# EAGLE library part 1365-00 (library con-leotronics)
DUAL ROW STRAIGHT HEADER 1364 SERIES. 1.27mm x 1.27mm. Without Fixing Post. SMT Source: http://www.leotronics.co.uk/Conexcon/Data%20Sheets/sec.%20A/1364ing.pdf
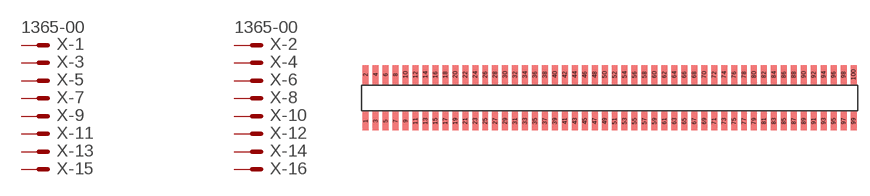
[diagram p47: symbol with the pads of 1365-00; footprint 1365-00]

Designator prefix X; gates -1=MVAL -2=MVAL -3=M -4=M -5=M -6=M -7=M -8=M -9=M -10=M -11=M -12=M -13=M -14=M -15=M -16=M -17=M -18=M -19=M -20=M -21=M -22=M -23=M -24=M -25=M -26=M -27=M -28=M -29=M -30=M -31=M -32=M -33=M -34=M -35=M -36=M -37=M -38=M -39=M -40=M -41=M -42=M -43=M -44=M -45=M -46=M -47=M -48=M -49=M -50=M -51=M -52=M -53=M -54=M -55=M -56=M -57=M -58=M -59=M -60=M -61=M -62=M -63=M -64=M -65=M -66=M -67=M -68=M -69=M -70=M -71=M -72=M -73=M -74=M -75=M -76=M -77=M -78=M -79=M -80=M -81=M -82=M -83=M -84=M -85=M -86=M -87=M -88=M -89=M -90=M -91=M -92=M -93=M -94=M -95=M -96=M -97=M -98=M -99=M -100=M

## 1365-00 (OC_FARNELL: unknown; OC_NEWARK: unknown)  [1365-00]
1  -1:S  pas
2  -2:S  pas
3  -3:S  pas
4  -4:S  pas
5  -5:S  pas
6  -6:S  pas
7  -7:S  pas
8  -8:S  pas
9  -9:S  pas
10  -10:S  pas
11  -11:S  pas
12  -12:S  pas
13  -13:S  pas
14  -14:S  pas
15  -15:S  pas
16  -16:S  pas
17  -17:S  pas
18  -18:S  pas
19  -19:S  pas
20  -20:S  pas
21  -21:S  pas
22  -22:S  pas
23  -23:S  pas
24  -24:S  pas
25  -25:S  pas
26  -26:S  pas
27  -27:S  pas
28  -28:S  pas
29  -29:S  pas
30  -30:S  pas
31  -31:S  pas
32  -32:S  pas
33  -33:S  pas
34  -34:S  pas
35  -35:S  pas
36  -36:S  pas
37  -37:S  pas
38  -38:S  pas
39  -39:S  pas
40  -40:S  pas
41  -41:S  pas
42  -42:S  pas
43  -43:S  pas
44  -44:S  pas
45  -45:S  pas
46  -46:S  pas
47  -47:S  pas
48  -48:S  pas
49  -49:S  pas
50  -50:S  pas
51  -51:S  pas
52  -52:S  pas
53  -53:S  pas
54  -54:S  pas
55  -55:S  pas
56  -56:S  pas
57  -57:S  pas
58  -58:S  pas
59  -59:S  pas
60  -60:S  pas
61  -61:S  pas
62  -62:S  pas
63  -63:S  pas
64  -64:S  pas
65  -65:S  pas
66  -66:S  pas
67  -67:S  pas
68  -68:S  pas
69  -69:S  pas
70  -70:S  pas
71  -71:S  pas
72  -72:S  pas
73  -73:S  pas
74  -74:S  pas
75  -75:S  pas
76  -76:S  pas
77  -77:S  pas
78  -78:S  pas
79  -79:S  pas
80  -80:S  pas
81  -81:S  pas
82  -82:S  pas
83  -83:S  pas
84  -84:S  pas
85  -85:S  pas
86  -86:S  pas
87  -87:S  pas
88  -88:S  pas
89  -89:S  pas
90  -90:S  pas
91  -91:S  pas
92  -92:S  pas
93  -93:S  pas
94  -94:S  pas
95  -95:S  pas
96  -96:S  pas
97  -97:S  pas
98  -98:S  pas
99  -99:S  pas
100  -100:S  pas

## Footprint 1365-00 (pad centres in mm)
DUAL ROW STRAIGHT HEADER 1364 SERIES. 1.27mm x 1.27mm. Without Fixing Post. SMT Source: http://www.leotronics.co.uk/Conexcon/Data%20Sheets/sec.%20A/1364ing.pdf
smd 0.76 x 2.4: 1 -31.115,-2.95; 2 -31.115,2.95; 3 -29.845,-2.95; 4 -29.845,2.95; 5 -28.575,-2.95; 6 -28.575,2.95; 7 -27.305,-2.95; 8 -27.305,2.95; 9 -26.035,-2.95; 10 -26.035,2.95; 11 -24.765,-2.95; 12 -24.765,2.95; 13 -23.495,-2.95; 14 -23.495,2.95; 15 -22.225,-2.95; 16 -22.225,2.95; 17 -20.955,-2.95; 18 -20.955,2.95; 19 -19.685,-2.95; 20 -19.685,2.95; 21 -18.415,-2.95; 22 -18.415,2.95; 23 -17.145,-2.95; 24 -17.145,2.95; 25 -15.875,-2.95; 26 -15.875,2.95; 27 -14.605,-2.95; 28 -14.605,2.95; 29 -13.335,-2.95; 30 -13.335,2.95; 31 -12.065,-2.95; 32 -12.065,2.95; 33 -10.795,-2.95; 34 -10.795,2.95; 35 -9.525,-2.95; 36 -9.525,2.95; 37 -8.255,-2.95; 38 -8.255,2.95; 39 -6.985,-2.95; 40 -6.985,2.95; 41 -5.715,-2.95; 42 -5.715,2.95; 43 -4.445,-2.95; 44 -4.445,2.95; 45 -3.175,-2.95; 46 -3.175,2.95; 47 -1.905,-2.95; 48 -1.905,2.95; 49 -0.635,-2.95; 50 -0.635,2.95; 51 0.635,-2.95; 52 0.635,2.95; 53 1.905,-2.95; 54 1.905,2.95; 55 3.175,-2.95; 56 3.175,2.95; 57 4.445,-2.95; 58 4.445,2.95; 59 5.715,-2.95; 60 5.715,2.95; 61 6.985,-2.95; 62 6.985,2.95; 63 8.255,-2.95; 64 8.255,2.95; 65 9.525,-2.95; 66 9.525,2.95; 67 10.795,-2.95; 68 10.795,2.95; 69 12.065,-2.95; 70 12.065,2.95; 71 13.335,-2.95; 72 13.335,2.95; 73 14.605,-2.95; 74 14.605,2.95; 75 15.875,-2.95; 76 15.875,2.95; 77 17.145,-2.95; 78 17.145,2.95; 79 18.415,-2.95; 80 18.415,2.95; 81 19.685,-2.95; 82 19.685,2.95; 83 20.955,-2.95; 84 20.955,2.95; 85 22.225,-2.95; 86 22.225,2.95; 87 23.495,-2.95; 88 23.495,2.95; 89 24.765,-2.95; 90 24.765,2.95; 91 26.035,-2.95; 92 26.035,2.95; 93 27.305,-2.95; 94 27.305,2.95; 95 28.575,-2.95; 96 28.575,2.95; 97 29.845,-2.95; 98 29.845,2.95; 99 31.115,-2.95; 100 31.115,2.95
